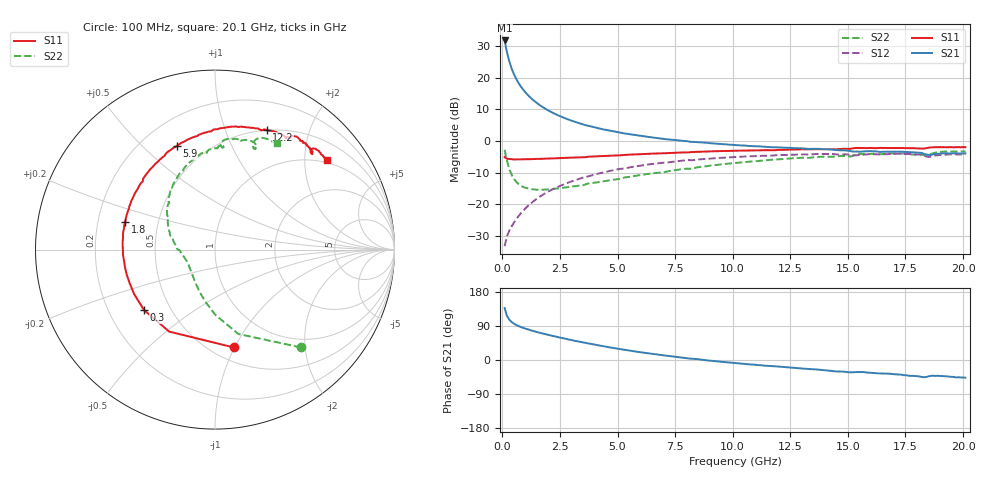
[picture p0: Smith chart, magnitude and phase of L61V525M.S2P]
!  Infineon Technologies AG
! BFR380L3 , PF131585-7, No.6, Th 09.10.01, soldered on pcb-board, measured with PP GSG850
!  Vce=1.5 V,  Ic=25.0 mA
! Common Emitter S-Parameters:  15. November 2001
#  GHz  S  MA  R  50
! f  S11  S21  S12  S22
! GHz  Mag  Ang  Mag  Ang  Mag  Ang  Mag  Ang
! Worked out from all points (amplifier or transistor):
!   201 points, 100 MHz to 20.1 GHz, reference 50 ohm
!   highest |S21| = 31.8 dB at 100 MHz (marker M1)
!   |S21| within 3 dB of that: start of sweep to 181.6 MHz
!   unconditionally stable (mu >= 1): 1.213 GHz to 4.53 GHz
!   at 3.4 GHz: K = 1.02, MAG = 7.8 dB, |S12| = -11.8 dB
!   at 10.1 GHz: K = 0.97, MSG = 1.9 dB, |S12| = -5.1 dB
!   at 20.1 GHz: K = 0.99, MSG = 0.1 dB, |S12| = -4.2 dB
!   S11 on the Smith chart (normalised r, x): 100 MHz: 0.63, -0.99; 300 MHz: 0.35, -0.33; 1.8 GHz: 0.32, +0.13; 5.9 GHz: 0.34, +0.64; 12.2 GHz: 0.49, +1.40; 20.1 GHz: 0.93, +2.56
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0.1  0.5555 -79.0  38.93 137.2  0.02169 58.9  0.7254 -48.7
0.2  0.5233 -119.2  25.5 116.7  0.03104 54.1  0.4879 -74.5
0.3  0.5193 -139.5  18.31 106.7  0.03795 54.8  0.3635 -89.7
0.4  0.5144 -151.1  14.15 100.4  0.04438 56.7  0.2947 -100.6
0.5  0.5109 -158.8  11.48 96.0  0.05076 59.1  0.2536 -109.2
0.6  0.5115 -164.7  9.646 92.6  0.05752 60.9  0.2272 -116.3
0.7  0.511 -169.6  8.328 89.7  0.06442 62.5  0.2094 -122.4
0.8  0.5108 -173.4  7.314 87.2  0.07151 63.5  0.1969 -127.6
1  0.513 -179.6  5.897 82.9  0.08585 64.8  0.1819 -136.1
1.2  0.5164 175.2  4.941 79.1  0.1002 65.2  0.1746 -142.8
1.5  0.5211 168.6  3.99 73.9  0.1222 65.0  0.1698 -150.6
1.8  0.5242 163.1  3.353 69.2  0.1442 64.1  0.17 -156.9
2.5  0.536 151.5  2.473 59.2  0.1942 60.7  0.1789 -167.9
3.5  0.5534 137.2  1.831 46.4  0.2634 54.2  0.1992 -179.5
4.6  0.5832 124.0  1.47 34.1  0.3323 46.6  0.2372 168.1
5.9  0.6161 110.2  1.223 21.3  0.4034 37.4  0.2858 155.0
6.8  0.6373 101.5  1.1 13.6  0.4465 30.8  0.3154 145.7
10.1  0.7013 77.4  0.8624 -8.0  0.5574 9.4  0.4493 118.7
12.2  0.7269 66.7  0.7854 -18.5  0.6015 -3.1  0.5211 102.8
13.5  0.7403 60.4  0.7533 -24.6  0.6162 -10.6  0.5513 94.2
16.8  0.7737 48.2  0.6806 -36.1  0.6206 -26.0  0.6325 74.9
20.1  0.798 38.6  0.6364 -46.6  0.6148 -39.3  0.6849 59.7
